DATA_BLOCK DB 101
TITLE =BLOCK DATA FOR TD_17 - OP_37
AUTHOR : Esposito
FAMILY : TEXER
NAME : BL_DAT1
VERSION : 0.1


  STRUCT
   W0 : ARRAY  [0 .. 100 ] OF //Word for start/stop at TD_17
   INT  := 0;
  END_STRUCT ;
BEGIN
   W0[0] := 2;
   W0[1] := 2;
   W0[2] := 0;
   W0[3] := 0;
   W0[4] := 0;
   W0[5] := 0;
   W0[6] := 11902;
   W0[7] := 0;
   W0[8] := 0;
   W0[9] := 0;
   W0[10] := 0;
   W0[11] := 0;
   W0[12] := 0;
   W0[13] := 0;
   W0[14] := 0;
   W0[15] := 0;
   W0[16] := 0;
   W0[17] := 0;
   W0[18] := 0;
   W0[19] := 0;
   W0[20] := 0;
   W0[21] := 0;
   W0[22] := 0;
   W0[23] := 0;
   W0[24] := 0;
   W0[25] := 0;
   W0[26] := 0;
   W0[27] := 0;
   W0[28] := 0;
   W0[29] := 0;
   W0[30] := 0;
   W0[31] := 0;
   W0[32] := 0;
   W0[33] := 0;
   W0[34] := 0;
   W0[35] := 0;
   W0[36] := 0;
   W0[37] := 0;
   W0[38] := 0;
   W0[39] := 0;
   W0[40] := 0;
   W0[41] := 0;
   W0[42] := 0;
   W0[43] := 0;
   W0[44] := 0;
   W0[45] := 0;
   W0[46] := 0;
   W0[47] := 0;
   W0[48] := 0;
   W0[49] := 0;
   W0[50] := 0;
   W0[51] := 0;
   W0[52] := 0;
   W0[53] := 0;
   W0[54] := 0;
   W0[55] := 0;
   W0[56] := 0;
   W0[57] := 0;
   W0[58] := 0;
   W0[59] := 0;
   W0[60] := 0;
   W0[61] := 0;
   W0[62] := 0;
   W0[63] := 0;
   W0[64] := 0;
   W0[65] := 0;
   W0[66] := 0;
   W0[67] := 0;
   W0[68] := 0;
   W0[69] := 0;
   W0[70] := 0;
   W0[71] := 0;
   W0[72] := 0;
   W0[73] := 0;
   W0[74] := 0;
   W0[75] := 0;
   W0[76] := 0;
   W0[77] := 0;
   W0[78] := 0;
   W0[79] := 0;
   W0[80] := 0;
   W0[81] := 0;
   W0[82] := 0;
   W0[83] := 0;
   W0[84] := 0;
   W0[85] := 0;
   W0[86] := 0;
   W0[87] := 0;
   W0[88] := 0;
   W0[89] := 0;
   W0[90] := 0;
   W0[91] := 0;
   W0[92] := 0;
   W0[93] := 0;
   W0[94] := 0;
   W0[95] := 0;
   W0[96] := 0;
   W0[97] := 0;
   W0[98] := 0;
   W0[99] := 0;
   W0[100] := 0;
END_DATA_BLOCK

